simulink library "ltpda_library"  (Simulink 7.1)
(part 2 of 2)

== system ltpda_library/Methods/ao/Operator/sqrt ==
  In1 : Inport  OutDataType=sfix(16)  OutScaling=2^0
  sqrt : M-S-Function  Tag=sqrt  FunctionName=ltpdasim
  Out1 : Outport  OutDataType=sfix(16)  OutScaling=2^0
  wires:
  In1/1 -> sqrt/1
  sqrt/1 -> Out1/1

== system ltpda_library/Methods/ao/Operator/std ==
  In1 : Inport  OutDataType=sfix(16)  OutScaling=2^0
  std : M-S-Function  Tag=std  FunctionName=ltpdasim
  Out1 : Outport  OutDataType=sfix(16)  OutScaling=2^0
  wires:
  In1/1 -> std/1
  std/1 -> Out1/1

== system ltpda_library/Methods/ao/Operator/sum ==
  In1 : Inport  OutDataType=sfix(16)  OutScaling=2^0
  sum : M-S-Function  Tag=sum  FunctionName=ltpdasim
  Out1 : Outport  OutDataType=sfix(16)  OutScaling=2^0
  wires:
  In1/1 -> sum/1
  sum/1 -> Out1/1

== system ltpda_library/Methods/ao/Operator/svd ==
  In1 : Inport  OutDataType=sfix(16)  OutScaling=2^0
  svd : M-S-Function  Tag=svd  FunctionName=ltpdasim
  Out1 : Outport  OutDataType=sfix(16)  OutScaling=2^0
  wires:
  In1/1 -> svd/1
  svd/1 -> Out1/1

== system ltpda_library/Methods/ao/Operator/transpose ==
  In1 : Inport  OutDataType=sfix(16)  OutScaling=2^0
  transpose : M-S-Function  Tag=transpose  FunctionName=ltpdasim
  Out1 : Outport  OutDataType=sfix(16)  OutScaling=2^0
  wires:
  In1/1 -> transpose/1
  transpose/1 -> Out1/1

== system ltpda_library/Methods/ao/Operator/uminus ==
  In1 : Inport  OutDataType=sfix(16)  OutScaling=2^0
  uminus : M-S-Function  Tag=uminus  FunctionName=ltpdasim
  Out1 : Outport  OutDataType=sfix(16)  OutScaling=2^0
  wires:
  In1/1 -> uminus/1
  uminus/1 -> Out1/1

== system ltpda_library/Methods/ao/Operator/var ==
  In1 : Inport  OutDataType=sfix(16)  OutScaling=2^0
  var : M-S-Function  Tag=var  FunctionName=ltpdasim
  Out1 : Outport  OutDataType=sfix(16)  OutScaling=2^0
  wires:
  In1/1 -> var/1
  var/1 -> Out1/1

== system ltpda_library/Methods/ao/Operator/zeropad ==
  In1 : Inport  OutDataType=sfix(16)  OutScaling=2^0
  zeropad : M-S-Function  Tag=zeropad  FunctionName=ltpdasim
  Out1 : Outport  OutDataType=sfix(16)  OutScaling=2^0
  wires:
  In1/1 -> zeropad/1
  zeropad/1 -> Out1/1

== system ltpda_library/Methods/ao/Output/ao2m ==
  In1 : Inport  OutDataType=sfix(16)  OutScaling=2^0
  Terminator : Terminator
  ao2m : M-S-Function  Tag=ao2m  FunctionName=ltpdasim
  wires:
  ao2m/1 -> Terminator/1
  In1/1 -> ao2m/1

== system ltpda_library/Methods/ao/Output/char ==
  In1 : Inport  OutDataType=sfix(16)  OutScaling=2^0
  Terminator : Terminator
  char : M-S-Function  Tag=char  FunctionName=ltpdasim
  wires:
  char/1 -> Terminator/1
  In1/1 -> char/1

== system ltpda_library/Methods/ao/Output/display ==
  In1 : Inport  OutDataType=sfix(16)  OutScaling=2^0
  Terminator : Terminator
  display : M-S-Function  Tag=display  FunctionName=ltpdasim
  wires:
  display/1 -> Terminator/1
  In1/1 -> display/1

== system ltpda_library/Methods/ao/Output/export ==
  In1 : Inport  OutDataType=sfix(16)  OutScaling=2^0
  Terminator : Terminator
  export : M-S-Function  Tag=export  FunctionName=ltpdasim
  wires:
  export/1 -> Terminator/1
  In1/1 -> export/1

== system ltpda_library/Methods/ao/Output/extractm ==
  In1 : Inport  OutDataType=sfix(16)  OutScaling=2^0
  Terminator : Terminator
  extractm : M-S-Function  Tag=extractm  FunctionName=ltpdasim
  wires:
  extractm/1 -> Terminator/1
  In1/1 -> extractm/1

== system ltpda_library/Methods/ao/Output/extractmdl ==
  In1 : Inport  OutDataType=sfix(16)  OutScaling=2^0
  Terminator : Terminator
  extractmdl : M-S-Function  Tag=extractmdl  FunctionName=ltpdasim
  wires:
  extractmdl/1 -> Terminator/1
  In1/1 -> extractmdl/1

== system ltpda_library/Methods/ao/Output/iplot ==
  In1 : Inport  OutDataType=sfix(16)  OutScaling=2^0
  Terminator : Terminator
  iplot : M-S-Function  Tag=iplot  FunctionName=ltpdasim
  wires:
  iplot/1 -> Terminator/1
  In1/1 -> iplot/1

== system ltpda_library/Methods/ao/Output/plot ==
  In1 : Inport  OutDataType=sfix(16)  OutScaling=2^0
  Terminator : Terminator
  plot : M-S-Function  Tag=plot  FunctionName=ltpdasim
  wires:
  plot/1 -> Terminator/1
  In1/1 -> plot/1

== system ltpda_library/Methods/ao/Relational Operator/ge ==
  In1 : Inport  OutDataType=sfix(16)  OutScaling=2^0
  ge : M-S-Function  Tag=ge  FunctionName=ltpdasim
  Out1 : Outport  OutDataType=sfix(16)  OutScaling=2^0
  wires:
  In1/1 -> ge/1
  ge/1 -> Out1/1

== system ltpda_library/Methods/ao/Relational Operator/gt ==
  In1 : Inport  OutDataType=sfix(16)  OutScaling=2^0
  gt : M-S-Function  Tag=gt  FunctionName=ltpdasim
  Out1 : Outport  OutDataType=sfix(16)  OutScaling=2^0
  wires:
  In1/1 -> gt/1
  gt/1 -> Out1/1

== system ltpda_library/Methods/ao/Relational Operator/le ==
  In1 : Inport  OutDataType=sfix(16)  OutScaling=2^0
  le : M-S-Function  Tag=le  FunctionName=ltpdasim
  Out1 : Outport  OutDataType=sfix(16)  OutScaling=2^0
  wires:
  In1/1 -> le/1
  le/1 -> Out1/1

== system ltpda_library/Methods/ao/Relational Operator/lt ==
  In1 : Inport  OutDataType=sfix(16)  OutScaling=2^0
  lt : M-S-Function  Tag=lt  FunctionName=ltpdasim
  Out1 : Outport  OutDataType=sfix(16)  OutScaling=2^0
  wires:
  In1/1 -> lt/1
  lt/1 -> Out1/1

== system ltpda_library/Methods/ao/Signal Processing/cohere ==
  In1 : Inport  OutDataType=sfix(16)  OutScaling=2^0
  cohere : M-S-Function  Tag=cohere  FunctionName=ltpdasim
  Out1 : Outport  OutDataType=sfix(16)  OutScaling=2^0
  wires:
  In1/1 -> cohere/1
  cohere/1 -> Out1/1

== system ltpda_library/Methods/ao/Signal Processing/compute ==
  In1 : Inport  OutDataType=sfix(16)  OutScaling=2^0
  compute : M-S-Function  Tag=compute  FunctionName=ltpdasim
  Out1 : Outport  OutDataType=sfix(16)  OutScaling=2^0
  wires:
  In1/1 -> compute/1
  compute/1 -> Out1/1

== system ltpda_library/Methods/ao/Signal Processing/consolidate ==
  In1 : Inport  OutDataType=sfix(16)  OutScaling=2^0
  consolidate : M-S-Function  Tag=consolidate  FunctionName=ltpdasim
  Out1 : Outport  OutDataType=sfix(16)  OutScaling=2^0
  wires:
  In1/1 -> consolidate/1
  consolidate/1 -> Out1/1

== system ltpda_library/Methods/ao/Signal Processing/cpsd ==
  In1 : Inport  OutDataType=sfix(16)  OutScaling=2^0
  cpsd : M-S-Function  Tag=cpsd  FunctionName=ltpdasim
  Out1 : Outport  OutDataType=sfix(16)  OutScaling=2^0
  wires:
  In1/1 -> cpsd/1
  cpsd/1 -> Out1/1

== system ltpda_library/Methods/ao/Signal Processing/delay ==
  In1 : Inport  OutDataType=sfix(16)  OutScaling=2^0
  delay : M-S-Function  Tag=delay  FunctionName=ltpdasim
  Out1 : Outport  OutDataType=sfix(16)  OutScaling=2^0
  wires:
  In1/1 -> delay/1
  delay/1 -> Out1/1

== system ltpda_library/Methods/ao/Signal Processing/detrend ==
  In1 : Inport  OutDataType=sfix(16)  OutScaling=2^0
  detrend : M-S-Function  Tag=detrend  FunctionName=ltpdasim
  Out1 : Outport  OutDataType=sfix(16)  OutScaling=2^0
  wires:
  In1/1 -> detrend/1
  detrend/1 -> Out1/1

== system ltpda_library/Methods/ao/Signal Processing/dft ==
  In1 : Inport  OutDataType=sfix(16)  OutScaling=2^0
  dft : M-S-Function  Tag=dft  FunctionName=ltpdasim
  Out1 : Outport  OutDataType=sfix(16)  OutScaling=2^0
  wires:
  In1/1 -> dft/1
  dft/1 -> Out1/1

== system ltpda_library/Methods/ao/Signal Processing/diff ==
  In1 : Inport  OutDataType=sfix(16)  OutScaling=2^0
  diff : M-S-Function  Tag=diff  FunctionName=ltpdasim
  Out1 : Outport  OutDataType=sfix(16)  OutScaling=2^0
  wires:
  In1/1 -> diff/1
  diff/1 -> Out1/1

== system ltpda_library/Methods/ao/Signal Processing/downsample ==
  In1 : Inport  OutDataType=sfix(16)  OutScaling=2^0
  downsample : M-S-Function  Tag=downsample  FunctionName=ltpdasim
  Out1 : Outport  OutDataType=sfix(16)  OutScaling=2^0
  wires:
  In1/1 -> downsample/1
  downsample/1 -> Out1/1

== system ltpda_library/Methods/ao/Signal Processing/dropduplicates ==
  In1 : Inport  OutDataType=sfix(16)  OutScaling=2^0
  dropduplicates : M-S-Function  Tag=dropduplicates  FunctionName=ltpdasim
  Out1 : Outport  OutDataType=sfix(16)  OutScaling=2^0
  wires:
  In1/1 -> dropduplicates/1
  dropduplicates/1 -> Out1/1

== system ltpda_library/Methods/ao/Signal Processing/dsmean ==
  In1 : Inport  OutDataType=sfix(16)  OutScaling=2^0
  dsmean : M-S-Function  Tag=dsmean  FunctionName=ltpdasim
  Out1 : Outport  OutDataType=sfix(16)  OutScaling=2^0
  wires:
  In1/1 -> dsmean/1
  dsmean/1 -> Out1/1

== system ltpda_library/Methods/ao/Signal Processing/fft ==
  In1 : Inport  OutDataType=sfix(16)  OutScaling=2^0
  fft : M-S-Function  Tag=fft  FunctionName=ltpdasim
  Out1 : Outport  OutDataType=sfix(16)  OutScaling=2^0
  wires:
  In1/1 -> fft/1
  fft/1 -> Out1/1

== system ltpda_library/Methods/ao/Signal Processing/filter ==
  In1 : Inport  OutDataType=sfix(16)  OutScaling=2^0
  filter : M-S-Function  Tag=filter  FunctionName=ltpdasim
  Out1 : Outport  OutDataType=sfix(16)  OutScaling=2^0
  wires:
  In1/1 -> filter/1
  filter/1 -> Out1/1

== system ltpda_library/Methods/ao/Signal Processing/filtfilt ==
  In1 : Inport  OutDataType=sfix(16)  OutScaling=2^0
  filtfilt : M-S-Function  Tag=filtfilt  FunctionName=ltpdasim
  Out1 : Outport  OutDataType=sfix(16)  OutScaling=2^0
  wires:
  In1/1 -> filtfilt/1
  filtfilt/1 -> Out1/1

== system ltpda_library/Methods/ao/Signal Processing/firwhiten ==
  In1 : Inport  OutDataType=sfix(16)  OutScaling=2^0
  firwhiten : M-S-Function  Tag=firwhiten  FunctionName=ltpdasim
  Out1 : Outport  OutDataType=sfix(16)  OutScaling=2^0
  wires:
  In1/1 -> firwhiten/1
  firwhiten/1 -> Out1/1

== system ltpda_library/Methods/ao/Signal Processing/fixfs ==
  In1 : Inport  OutDataType=sfix(16)  OutScaling=2^0
  fixfs : M-S-Function  Tag=fixfs  FunctionName=ltpdasim
  Out1 : Outport  OutDataType=sfix(16)  OutScaling=2^0
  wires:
  In1/1 -> fixfs/1
  fixfs/1 -> Out1/1

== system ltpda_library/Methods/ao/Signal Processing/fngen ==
  In1 : Inport  OutDataType=sfix(16)  OutScaling=2^0
  fngen : M-S-Function  Tag=fngen  FunctionName=ltpdasim
  Out1 : Outport  OutDataType=sfix(16)  OutScaling=2^0
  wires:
  In1/1 -> fngen/1
  fngen/1 -> Out1/1

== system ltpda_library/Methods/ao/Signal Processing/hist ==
  In1 : Inport  OutDataType=sfix(16)  OutScaling=2^0
  hist : M-S-Function  Tag=hist  FunctionName=ltpdasim
  Out1 : Outport  OutDataType=sfix(16)  OutScaling=2^0
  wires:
  In1/1 -> hist/1
  hist/1 -> Out1/1

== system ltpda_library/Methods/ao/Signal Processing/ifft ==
  In1 : Inport  OutDataType=sfix(16)  OutScaling=2^0
  ifft : M-S-Function  Tag=ifft  FunctionName=ltpdasim
  Out1 : Outport  OutDataType=sfix(16)  OutScaling=2^0
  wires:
  In1/1 -> ifft/1
  ifft/1 -> Out1/1

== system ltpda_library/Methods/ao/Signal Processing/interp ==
  In1 : Inport  OutDataType=sfix(16)  OutScaling=2^0
  interp : M-S-Function  Tag=interp  FunctionName=ltpdasim
  Out1 : Outport  OutDataType=sfix(16)  OutScaling=2^0
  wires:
  In1/1 -> interp/1
  interp/1 -> Out1/1

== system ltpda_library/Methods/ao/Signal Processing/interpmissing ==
  In1 : Inport  OutDataType=sfix(16)  OutScaling=2^0
  interpmissing : M-S-Function  Tag=interpmissing  FunctionName=ltpdasim
  Out1 : Outport  OutDataType=sfix(16)  OutScaling=2^0
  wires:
  In1/1 -> interpmissing/1
  interpmissing/1 -> Out1/1

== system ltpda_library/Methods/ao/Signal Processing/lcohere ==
  In1 : Inport  OutDataType=sfix(16)  OutScaling=2^0
  lcohere : M-S-Function  Tag=lcohere  FunctionName=ltpdasim
  Out1 : Outport  OutDataType=sfix(16)  OutScaling=2^0
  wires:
  In1/1 -> lcohere/1
  lcohere/1 -> Out1/1

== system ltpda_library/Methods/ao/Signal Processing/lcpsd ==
  In1 : Inport  OutDataType=sfix(16)  OutScaling=2^0
  lcpsd : M-S-Function  Tag=lcpsd  FunctionName=ltpdasim
  Out1 : Outport  OutDataType=sfix(16)  OutScaling=2^0
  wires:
  In1/1 -> lcpsd/1
  lcpsd/1 -> Out1/1

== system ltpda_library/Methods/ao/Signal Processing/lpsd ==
  In1 : Inport  OutDataType=sfix(16)  OutScaling=2^0
  lpsd : M-S-Function  Tag=lpsd  FunctionName=ltpdasim
  Out1 : Outport  OutDataType=sfix(16)  OutScaling=2^0
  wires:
  In1/1 -> lpsd/1
  lpsd/1 -> Out1/1

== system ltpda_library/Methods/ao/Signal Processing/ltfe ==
  In1 : Inport  OutDataType=sfix(16)  OutScaling=2^0
  ltfe : M-S-Function  Tag=ltfe  FunctionName=ltpdasim
  Out1 : Outport  OutDataType=sfix(16)  OutScaling=2^0
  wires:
  In1/1 -> ltfe/1
  ltfe/1 -> Out1/1

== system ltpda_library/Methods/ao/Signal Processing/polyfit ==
  In1 : Inport  OutDataType=sfix(16)  OutScaling=2^0
  polyfit : M-S-Function  Tag=polyfit  FunctionName=ltpdasim
  Out1 : Outport  OutDataType=sfix(16)  OutScaling=2^0
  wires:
  In1/1 -> polyfit/1
  polyfit/1 -> Out1/1

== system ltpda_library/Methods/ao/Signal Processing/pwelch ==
  In1 : Inport  OutDataType=sfix(16)  OutScaling=2^0
  pwelch : M-S-Function  Tag=pwelch  FunctionName=ltpdasim
  Out1 : Outport  OutDataType=sfix(16)  OutScaling=2^0
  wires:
  In1/1 -> pwelch/1
  pwelch/1 -> Out1/1

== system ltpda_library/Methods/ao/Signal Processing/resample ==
  In1 : Inport  OutDataType=sfix(16)  OutScaling=2^0
  resample : M-S-Function  Tag=resample  FunctionName=ltpdasim
  Out1 : Outport  OutDataType=sfix(16)  OutScaling=2^0
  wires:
  In1/1 -> resample/1
  resample/1 -> Out1/1

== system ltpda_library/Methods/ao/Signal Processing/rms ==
  In1 : Inport  OutDataType=sfix(16)  OutScaling=2^0
  rms : M-S-Function  Tag=rms  FunctionName=ltpdasim
  Out1 : Outport  OutDataType=sfix(16)  OutScaling=2^0
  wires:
  In1/1 -> rms/1
  rms/1 -> Out1/1

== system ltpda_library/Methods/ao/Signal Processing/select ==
  In1 : Inport  OutDataType=sfix(16)  OutScaling=2^0
  select : M-S-Function  Tag=select  FunctionName=ltpdasim
  Out1 : Outport  OutDataType=sfix(16)  OutScaling=2^0
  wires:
  In1/1 -> select/1
  select/1 -> Out1/1

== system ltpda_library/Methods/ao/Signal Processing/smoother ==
  In1 : Inport  OutDataType=sfix(16)  OutScaling=2^0
  smoother : M-S-Function  Tag=smoother  FunctionName=ltpdasim
  Out1 : Outport  OutDataType=sfix(16)  OutScaling=2^0
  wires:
  In1/1 -> smoother/1
  smoother/1 -> Out1/1

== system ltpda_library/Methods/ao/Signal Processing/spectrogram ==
  In1 : Inport  OutDataType=sfix(16)  OutScaling=2^0
  spectrogram : M-S-Function  Tag=spectrogram  FunctionName=ltpdasim
  Out1 : Outport  OutDataType=sfix(16)  OutScaling=2^0
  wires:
  In1/1 -> spectrogram/1
  spectrogram/1 -> Out1/1

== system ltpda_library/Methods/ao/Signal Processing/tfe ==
  In1 : Inport  OutDataType=sfix(16)  OutScaling=2^0
  tfe : M-S-Function  Tag=tfe  FunctionName=ltpdasim
  Out1 : Outport  OutDataType=sfix(16)  OutScaling=2^0
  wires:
  In1/1 -> tfe/1
  tfe/1 -> Out1/1

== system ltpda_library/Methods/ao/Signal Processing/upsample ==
  In1 : Inport  OutDataType=sfix(16)  OutScaling=2^0
  upsample : M-S-Function  Tag=upsample  FunctionName=ltpdasim
  Out1 : Outport  OutDataType=sfix(16)  OutScaling=2^0
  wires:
  In1/1 -> upsample/1
  upsample/1 -> Out1/1

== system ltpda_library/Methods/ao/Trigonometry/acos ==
  In1 : Inport  OutDataType=sfix(16)  OutScaling=2^0
  acos : M-S-Function  Tag=acos  FunctionName=ltpdasim
  Out1 : Outport  OutDataType=sfix(16)  OutScaling=2^0
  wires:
  In1/1 -> acos/1
  acos/1 -> Out1/1

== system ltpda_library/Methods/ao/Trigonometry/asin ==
  In1 : Inport  OutDataType=sfix(16)  OutScaling=2^0
  asin : M-S-Function  Tag=asin  FunctionName=ltpdasim
  Out1 : Outport  OutDataType=sfix(16)  OutScaling=2^0
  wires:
  In1/1 -> asin/1
  asin/1 -> Out1/1

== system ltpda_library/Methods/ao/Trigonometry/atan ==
  In1 : Inport  OutDataType=sfix(16)  OutScaling=2^0
  atan : M-S-Function  Tag=atan  FunctionName=ltpdasim
  Out1 : Outport  OutDataType=sfix(16)  OutScaling=2^0
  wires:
  In1/1 -> atan/1
  atan/1 -> Out1/1

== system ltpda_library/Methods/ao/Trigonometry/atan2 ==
  In1 : Inport  OutDataType=sfix(16)  OutScaling=2^0
  atan2 : M-S-Function  Tag=atan2  FunctionName=ltpdasim
  Out1 : Outport  OutDataType=sfix(16)  OutScaling=2^0
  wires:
  In1/1 -> atan2/1
  atan2/1 -> Out1/1

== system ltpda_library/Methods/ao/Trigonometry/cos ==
  In1 : Inport  OutDataType=sfix(16)  OutScaling=2^0
  cos : M-S-Function  Tag=cos  FunctionName=ltpdasim
  Out1 : Outport  OutDataType=sfix(16)  OutScaling=2^0
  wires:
  In1/1 -> cos/1
  cos/1 -> Out1/1

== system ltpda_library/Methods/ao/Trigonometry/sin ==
  In1 : Inport  OutDataType=sfix(16)  OutScaling=2^0
  sin : M-S-Function  Tag=sin  FunctionName=ltpdasim
  Out1 : Outport  OutDataType=sfix(16)  OutScaling=2^0
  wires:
  In1/1 -> sin/1
  sin/1 -> Out1/1

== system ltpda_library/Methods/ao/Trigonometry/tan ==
  In1 : Inport  OutDataType=sfix(16)  OutScaling=2^0
  tan : M-S-Function  Tag=tan  FunctionName=ltpdasim
  Out1 : Outport  OutDataType=sfix(16)  OutScaling=2^0
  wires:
  In1/1 -> tan/1
  tan/1 -> Out1/1

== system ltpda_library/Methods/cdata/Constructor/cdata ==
  Ground : Ground
  cdata : M-S-Function  Tag=cdata  FunctionName=ltpdasim
  Out1 : Outport  OutDataType=sfix(16)  OutScaling=2^0
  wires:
  Ground/1 -> cdata/1
  cdata/1 -> Out1/1

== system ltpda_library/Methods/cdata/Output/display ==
  In1 : Inport  OutDataType=sfix(16)  OutScaling=2^0
  Terminator : Terminator
  display : M-S-Function  Tag=display  FunctionName=ltpdasim
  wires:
  display/1 -> Terminator/1
  In1/1 -> display/1

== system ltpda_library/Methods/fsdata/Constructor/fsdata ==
  Ground : Ground
  fsdata : M-S-Function  Tag=fsdata  FunctionName=ltpdasim
  Out1 : Outport  OutDataType=sfix(16)  OutScaling=2^0
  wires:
  Ground/1 -> fsdata/1
  fsdata/1 -> Out1/1

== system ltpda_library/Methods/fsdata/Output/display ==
  In1 : Inport  OutDataType=sfix(16)  OutScaling=2^0
  Terminator : Terminator
  display : M-S-Function  Tag=display  FunctionName=ltpdasim
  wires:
  display/1 -> Terminator/1
  In1/1 -> display/1

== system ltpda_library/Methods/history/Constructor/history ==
  Ground : Ground
  history : M-S-Function  Tag=history  FunctionName=ltpdasim
  Out1 : Outport  OutDataType=sfix(16)  OutScaling=2^0
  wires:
  Ground/1 -> history/1
  history/1 -> Out1/1

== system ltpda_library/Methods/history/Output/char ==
  In1 : Inport  OutDataType=sfix(16)  OutScaling=2^0
  Terminator : Terminator
  char : M-S-Function  Tag=char  FunctionName=ltpdasim
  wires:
  char/1 -> Terminator/1
  In1/1 -> char/1

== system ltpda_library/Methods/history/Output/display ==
  In1 : Inport  OutDataType=sfix(16)  OutScaling=2^0
  Terminator : Terminator
  display : M-S-Function  Tag=display  FunctionName=ltpdasim
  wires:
  display/1 -> Terminator/1
  In1/1 -> display/1

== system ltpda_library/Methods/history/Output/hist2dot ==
  In1 : Inport  OutDataType=sfix(16)  OutScaling=2^0
  Terminator : Terminator
  hist2dot : M-S-Function  Tag=hist2dot  FunctionName=ltpdasim
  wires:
  hist2dot/1 -> Terminator/1
  In1/1 -> hist2dot/1

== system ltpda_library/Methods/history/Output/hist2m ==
  In1 : Inport  OutDataType=sfix(16)  OutScaling=2^0
  Terminator : Terminator
  hist2m : M-S-Function  Tag=hist2m  FunctionName=ltpdasim
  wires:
  hist2m/1 -> Terminator/1
  In1/1 -> hist2m/1

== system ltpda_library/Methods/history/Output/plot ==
  In1 : Inport  OutDataType=sfix(16)  OutScaling=2^0
  Terminator : Terminator
  plot : M-S-Function  Tag=plot  FunctionName=ltpdasim
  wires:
  plot/1 -> Terminator/1
  In1/1 -> plot/1

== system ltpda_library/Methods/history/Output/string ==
  In1 : Inport  OutDataType=sfix(16)  OutScaling=2^0
  Terminator : Terminator
  string : M-S-Function  Tag=string  FunctionName=ltpdasim
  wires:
  string/1 -> Terminator/1
  In1/1 -> string/1

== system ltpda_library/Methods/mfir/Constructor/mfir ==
  Ground : Ground
  mfir : M-S-Function  Tag=mfir  FunctionName=ltpdasim
  Out1 : Outport  OutDataType=sfix(16)  OutScaling=2^0
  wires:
  Ground/1 -> mfir/1
  mfir/1 -> Out1/1

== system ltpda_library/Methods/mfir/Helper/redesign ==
  In1 : Inport  OutDataType=sfix(16)  OutScaling=2^0
  redesign : M-S-Function  Tag=redesign  FunctionName=ltpdasim
  Out1 : Outport  OutDataType=sfix(16)  OutScaling=2^0
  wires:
  In1/1 -> redesign/1
  redesign/1 -> Out1/1

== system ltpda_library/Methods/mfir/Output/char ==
  In1 : Inport  OutDataType=sfix(16)  OutScaling=2^0
  Terminator : Terminator
  char : M-S-Function  Tag=char  FunctionName=ltpdasim
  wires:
  char/1 -> Terminator/1
  In1/1 -> char/1

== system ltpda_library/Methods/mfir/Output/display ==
  In1 : Inport  OutDataType=sfix(16)  OutScaling=2^0
  Terminator : Terminator
  display : M-S-Function  Tag=display  FunctionName=ltpdasim
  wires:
  display/1 -> Terminator/1
  In1/1 -> display/1

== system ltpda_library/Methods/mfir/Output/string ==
  In1 : Inport  OutDataType=sfix(16)  OutScaling=2^0
  Terminator : Terminator
  string : M-S-Function  Tag=string  FunctionName=ltpdasim
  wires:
  string/1 -> Terminator/1
  In1/1 -> string/1

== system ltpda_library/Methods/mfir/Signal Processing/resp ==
  In1 : Inport  OutDataType=sfix(16)  OutScaling=2^0
  resp : M-S-Function  Tag=resp  FunctionName=ltpdasim
  Out1 : Outport  OutDataType=sfix(16)  OutScaling=2^0
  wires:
  In1/1 -> resp/1
  resp/1 -> Out1/1

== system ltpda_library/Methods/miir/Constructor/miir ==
  Ground : Ground
  miir : M-S-Function  Tag=miir  FunctionName=ltpdasim
  Out1 : Outport  OutDataType=sfix(16)  OutScaling=2^0
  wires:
  Ground/1 -> miir/1
  miir/1 -> Out1/1

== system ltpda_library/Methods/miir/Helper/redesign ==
  In1 : Inport  OutDataType=sfix(16)  OutScaling=2^0
  redesign : M-S-Function  Tag=redesign  FunctionName=ltpdasim
  Out1 : Outport  OutDataType=sfix(16)  OutScaling=2^0
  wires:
  In1/1 -> redesign/1
  redesign/1 -> Out1/1

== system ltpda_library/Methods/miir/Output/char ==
  In1 : Inport  OutDataType=sfix(16)  OutScaling=2^0
  Terminator : Terminator
  char : M-S-Function  Tag=char  FunctionName=ltpdasim
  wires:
  char/1 -> Terminator/1
  In1/1 -> char/1

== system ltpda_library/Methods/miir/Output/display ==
  In1 : Inport  OutDataType=sfix(16)  OutScaling=2^0
  Terminator : Terminator
  display : M-S-Function  Tag=display  FunctionName=ltpdasim
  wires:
  display/1 -> Terminator/1
  In1/1 -> display/1

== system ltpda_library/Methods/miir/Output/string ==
  In1 : Inport  OutDataType=sfix(16)  OutScaling=2^0
  Terminator : Terminator
  string : M-S-Function  Tag=string  FunctionName=ltpdasim
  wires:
  string/1 -> Terminator/1
  In1/1 -> string/1

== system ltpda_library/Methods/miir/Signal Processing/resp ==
  In1 : Inport  OutDataType=sfix(16)  OutScaling=2^0
  resp : M-S-Function  Tag=resp  FunctionName=ltpdasim
  Out1 : Outport  OutDataType=sfix(16)  OutScaling=2^0
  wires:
  In1/1 -> resp/1
  resp/1 -> Out1/1

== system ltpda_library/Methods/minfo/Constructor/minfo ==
  Ground : Ground
  minfo : M-S-Function  Tag=minfo  FunctionName=ltpdasim
  Out1 : Outport  OutDataType=sfix(16)  OutScaling=2^0
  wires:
  Ground/1 -> minfo/1
  minfo/1 -> Out1/1

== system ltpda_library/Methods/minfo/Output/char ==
  In1 : Inport  OutDataType=sfix(16)  OutScaling=2^0
  Terminator : Terminator
  char : M-S-Function  Tag=char  FunctionName=ltpdasim
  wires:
  char/1 -> Terminator/1
  In1/1 -> char/1

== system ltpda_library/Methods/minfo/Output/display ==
  In1 : Inport  OutDataType=sfix(16)  OutScaling=2^0
  Terminator : Terminator
  display : M-S-Function  Tag=display  FunctionName=ltpdasim
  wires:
  display/1 -> Terminator/1
  In1/1 -> display/1

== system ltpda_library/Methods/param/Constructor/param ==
  Ground : Ground
  param : M-S-Function  Tag=param  FunctionName=ltpdasim
  Out1 : Outport  OutDataType=sfix(16)  OutScaling=2^0
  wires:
  Ground/1 -> param/1
  param/1 -> Out1/1

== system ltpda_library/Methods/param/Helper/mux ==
  In1 : Inport  OutDataType=sfix(16)  OutScaling=2^0
  mux : M-S-Function  Tag=mux  FunctionName=ltpdasim
  Out1 : Outport  OutDataType=sfix(16)  OutScaling=2^0
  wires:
  In1/1 -> mux/1
  mux/1 -> Out1/1

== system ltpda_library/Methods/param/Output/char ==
  In1 : Inport  OutDataType=sfix(16)  OutScaling=2^0
  Terminator : Terminator
  char : M-S-Function  Tag=char  FunctionName=ltpdasim
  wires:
  char/1 -> Terminator/1
  In1/1 -> char/1

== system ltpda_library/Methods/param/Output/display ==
  In1 : Inport  OutDataType=sfix(16)  OutScaling=2^0
  Terminator : Terminator
  display : M-S-Function  Tag=display  FunctionName=ltpdasim
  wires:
  display/1 -> Terminator/1
  In1/1 -> display/1

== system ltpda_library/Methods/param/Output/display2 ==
  In1 : Inport  OutDataType=sfix(16)  OutScaling=2^0
  Terminator : Terminator
  display2 : M-S-Function  Tag=display2  FunctionName=ltpdasim
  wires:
  display2/1 -> Terminator/1
  In1/1 -> display2/1

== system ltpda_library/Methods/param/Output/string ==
  In1 : Inport  OutDataType=sfix(16)  OutScaling=2^0
  Terminator : Terminator
  string : M-S-Function  Tag=string  FunctionName=ltpdasim
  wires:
  string/1 -> Terminator/1
  In1/1 -> string/1

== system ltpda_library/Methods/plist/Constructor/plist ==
  Ground : Ground
  plist : M-S-Function  Tag=plist  FunctionName=ltpdasim
  Out1 : Outport  OutDataType=sfix(16)  OutScaling=2^0
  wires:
  Ground/1 -> plist/1
  plist/1 -> Out1/1

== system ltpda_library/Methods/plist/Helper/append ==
  In1 : Inport  OutDataType=sfix(16)  OutScaling=2^0
  append : M-S-Function  Tag=append  FunctionName=ltpdasim
  Out1 : Outport  OutDataType=sfix(16)  OutScaling=2^0
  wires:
  In1/1 -> append/1
  append/1 -> Out1/1

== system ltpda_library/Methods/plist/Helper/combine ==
  In1 : Inport  OutDataType=sfix(16)  OutScaling=2^0
  combine : M-S-Function  Tag=combine  FunctionName=ltpdasim
  Out1 : Outport  OutDataType=sfix(16)  OutScaling=2^0
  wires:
  In1/1 -> combine/1
  combine/1 -> Out1/1

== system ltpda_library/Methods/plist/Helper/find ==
  In1 : Inport  OutDataType=sfix(16)  OutScaling=2^0
  find : M-S-Function  Tag=find  FunctionName=ltpdasim
  Out1 : Outport  OutDataType=sfix(16)  OutScaling=2^0
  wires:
  In1/1 -> find/1
  find/1 -> Out1/1

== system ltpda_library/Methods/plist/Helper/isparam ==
  In1 : Inport  OutDataType=sfix(16)  OutScaling=2^0
  isparam : M-S-Function  Tag=isparam  FunctionName=ltpdasim
  Out1 : Outport  OutDataType=sfix(16)  OutScaling=2^0
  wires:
  In1/1 -> isparam/1
  isparam/1 -> Out1/1

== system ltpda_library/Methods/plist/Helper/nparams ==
  In1 : Inport  OutDataType=sfix(16)  OutScaling=2^0
  nparams : M-S-Function  Tag=nparams  FunctionName=ltpdasim
  Out1 : Outport  OutDataType=sfix(16)  OutScaling=2^0
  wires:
  In1/1 -> nparams/1
  nparams/1 -> Out1/1

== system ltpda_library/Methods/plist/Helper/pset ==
  In1 : Inport  OutDataType=sfix(16)  OutScaling=2^0
  pset : M-S-Function  Tag=pset  FunctionName=ltpdasim
  Out1 : Outport  OutDataType=sfix(16)  OutScaling=2^0
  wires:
  In1/1 -> pset/1
  pset/1 -> Out1/1

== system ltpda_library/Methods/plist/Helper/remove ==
  In1 : Inport  OutDataType=sfix(16)  OutScaling=2^0
  remove : M-S-Function  Tag=remove  FunctionName=ltpdasim
  Out1 : Outport  OutDataType=sfix(16)  OutScaling=2^0
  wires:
  In1/1 -> remove/1
  remove/1 -> Out1/1

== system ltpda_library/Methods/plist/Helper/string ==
  In1 : Inport  OutDataType=sfix(16)  OutScaling=2^0
  string : M-S-Function  Tag=string  FunctionName=ltpdasim
  Out1 : Outport  OutDataType=sfix(16)  OutScaling=2^0
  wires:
  In1/1 -> string/1
  string/1 -> Out1/1

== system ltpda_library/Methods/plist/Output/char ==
  In1 : Inport  OutDataType=sfix(16)  OutScaling=2^0
  Terminator : Terminator
  char : M-S-Function  Tag=char  FunctionName=ltpdasim
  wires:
  char/1 -> Terminator/1
  In1/1 -> char/1

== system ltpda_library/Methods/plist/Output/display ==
  In1 : Inport  OutDataType=sfix(16)  OutScaling=2^0
  Terminator : Terminator
  display : M-S-Function  Tag=display  FunctionName=ltpdasim
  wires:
  display/1 -> Terminator/1
  In1/1 -> display/1

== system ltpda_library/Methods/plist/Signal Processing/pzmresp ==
  In1 : Inport  OutDataType=sfix(16)  OutScaling=2^0
  pzmresp : M-S-Function  Tag=pzmresp  FunctionName=ltpdasim
  Out1 : Outport  OutDataType=sfix(16)  OutScaling=2^0
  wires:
  In1/1 -> pzmresp/1
  pzmresp/1 -> Out1/1

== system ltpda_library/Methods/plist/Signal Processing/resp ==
  In1 : Inport  OutDataType=sfix(16)  OutScaling=2^0
  resp : M-S-Function  Tag=resp  FunctionName=ltpdasim
  Out1 : Outport  OutDataType=sfix(16)  OutScaling=2^0
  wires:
  In1/1 -> resp/1
  resp/1 -> Out1/1

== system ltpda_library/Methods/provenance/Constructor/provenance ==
  Ground : Ground
  provenance : M-S-Function  Tag=provenance  FunctionName=ltpdasim
  Out1 : Outport  OutDataType=sfix(16)  OutScaling=2^0
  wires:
  Ground/1 -> provenance/1
  provenance/1 -> Out1/1

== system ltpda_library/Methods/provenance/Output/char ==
  In1 : Inport  OutDataType=sfix(16)  OutScaling=2^0
  Terminator : Terminator
  char : M-S-Function  Tag=char  FunctionName=ltpdasim
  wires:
  char/1 -> Terminator/1
  In1/1 -> char/1

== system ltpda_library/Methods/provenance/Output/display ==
  In1 : Inport  OutDataType=sfix(16)  OutScaling=2^0
  Terminator : Terminator
  display : M-S-Function  Tag=display  FunctionName=ltpdasim
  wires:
  display/1 -> Terminator/1
  In1/1 -> display/1

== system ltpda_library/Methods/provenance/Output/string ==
  In1 : Inport  OutDataType=sfix(16)  OutScaling=2^0
  Terminator : Terminator
  string : M-S-Function  Tag=string  FunctionName=ltpdasim
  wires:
  string/1 -> Terminator/1
  In1/1 -> string/1

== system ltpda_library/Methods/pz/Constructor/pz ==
  Ground : Ground
  pz : M-S-Function  Tag=pz  FunctionName=ltpdasim
  Out1 : Outport  OutDataType=sfix(16)  OutScaling=2^0
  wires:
  Ground/1 -> pz/1
  pz/1 -> Out1/1

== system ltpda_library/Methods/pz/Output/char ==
  In1 : Inport  OutDataType=sfix(16)  OutScaling=2^0
  Terminator : Terminator
  char : M-S-Function  Tag=char  FunctionName=ltpdasim
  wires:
  char/1 -> Terminator/1
  In1/1 -> char/1

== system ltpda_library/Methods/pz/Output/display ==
  In1 : Inport  OutDataType=sfix(16)  OutScaling=2^0
  Terminator : Terminator
  display : M-S-Function  Tag=display  FunctionName=ltpdasim
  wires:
  display/1 -> Terminator/1
  In1/1 -> display/1

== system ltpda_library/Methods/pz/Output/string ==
  In1 : Inport  OutDataType=sfix(16)  OutScaling=2^0
  Terminator : Terminator
  string : M-S-Function  Tag=string  FunctionName=ltpdasim
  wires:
  string/1 -> Terminator/1
  In1/1 -> string/1

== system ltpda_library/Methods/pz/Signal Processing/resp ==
  In1 : Inport  OutDataType=sfix(16)  OutScaling=2^0
  resp : M-S-Function  Tag=resp  FunctionName=ltpdasim
  Out1 : Outport  OutDataType=sfix(16)  OutScaling=2^0
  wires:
  In1/1 -> resp/1
  resp/1 -> Out1/1

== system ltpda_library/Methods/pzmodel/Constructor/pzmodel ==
  Ground : Ground
  pzmodel : M-S-Function  Tag=pzmodel  FunctionName=ltpdasim
  Out1 : Outport  OutDataType=sfix(16)  OutScaling=2^0
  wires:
  Ground/1 -> pzmodel/1
  pzmodel/1 -> Out1/1

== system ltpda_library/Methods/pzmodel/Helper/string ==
  In1 : Inport  OutDataType=sfix(16)  OutScaling=2^0
  string : M-S-Function  Tag=string  FunctionName=ltpdasim
  Out1 : Outport  OutDataType=sfix(16)  OutScaling=2^0
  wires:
  In1/1 -> string/1
  string/1 -> Out1/1

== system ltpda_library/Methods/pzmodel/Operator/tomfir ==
  In1 : Inport  OutDataType=sfix(16)  OutScaling=2^0
  tomfir : M-S-Function  Tag=tomfir  FunctionName=ltpdasim
  Out1 : Outport  OutDataType=sfix(16)  OutScaling=2^0
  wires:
  In1/1 -> tomfir/1
  tomfir/1 -> Out1/1

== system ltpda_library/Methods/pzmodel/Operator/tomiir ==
  In1 : Inport  OutDataType=sfix(16)  OutScaling=2^0
  tomiir : M-S-Function  Tag=tomiir  FunctionName=ltpdasim
  Out1 : Outport  OutDataType=sfix(16)  OutScaling=2^0
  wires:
  In1/1 -> tomiir/1
  tomiir/1 -> Out1/1

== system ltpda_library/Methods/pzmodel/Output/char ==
  In1 : Inport  OutDataType=sfix(16)  OutScaling=2^0
  Terminator : Terminator
  char : M-S-Function  Tag=char  FunctionName=ltpdasim
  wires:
  char/1 -> Terminator/1
  In1/1 -> char/1

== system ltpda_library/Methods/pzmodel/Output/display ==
  In1 : Inport  OutDataType=sfix(16)  OutScaling=2^0
  Terminator : Terminator
  display : M-S-Function  Tag=display  FunctionName=ltpdasim
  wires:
  display/1 -> Terminator/1
  In1/1 -> display/1

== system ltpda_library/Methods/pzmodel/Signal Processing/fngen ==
  In1 : Inport  OutDataType=sfix(16)  OutScaling=2^0
  fngen : M-S-Function  Tag=fngen  FunctionName=ltpdasim
  Out1 : Outport  OutDataType=sfix(16)  OutScaling=2^0
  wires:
  In1/1 -> fngen/1
  fngen/1 -> Out1/1

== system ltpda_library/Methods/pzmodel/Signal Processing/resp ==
  In1 : Inport  OutDataType=sfix(16)  OutScaling=2^0
  resp : M-S-Function  Tag=resp  FunctionName=ltpdasim
  Out1 : Outport  OutDataType=sfix(16)  OutScaling=2^0
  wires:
  In1/1 -> resp/1
  resp/1 -> Out1/1

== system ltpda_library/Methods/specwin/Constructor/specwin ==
  Ground : Ground
  specwin : M-S-Function  Tag=specwin  FunctionName=ltpdasim
  Out1 : Outport  OutDataType=sfix(16)  OutScaling=2^0
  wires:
  Ground/1 -> specwin/1
  specwin/1 -> Out1/1

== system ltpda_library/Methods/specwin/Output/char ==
  In1 : Inport  OutDataType=sfix(16)  OutScaling=2^0
  Terminator : Terminator
  char : M-S-Function  Tag=char  FunctionName=ltpdasim
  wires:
  char/1 -> Terminator/1
  In1/1 -> char/1

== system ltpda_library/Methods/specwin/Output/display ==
  In1 : Inport  OutDataType=sfix(16)  OutScaling=2^0
  Terminator : Terminator
  display : M-S-Function  Tag=display  FunctionName=ltpdasim
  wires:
  display/1 -> Terminator/1
  In1/1 -> display/1

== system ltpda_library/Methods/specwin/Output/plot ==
  In1 : Inport  OutDataType=sfix(16)  OutScaling=2^0
  Terminator : Terminator
  plot : M-S-Function  Tag=plot  FunctionName=ltpdasim
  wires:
  plot/1 -> Terminator/1
  In1/1 -> plot/1

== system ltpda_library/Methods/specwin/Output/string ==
  In1 : Inport  OutDataType=sfix(16)  OutScaling=2^0
  Terminator : Terminator
  string : M-S-Function  Tag=string  FunctionName=ltpdasim
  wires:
  string/1 -> Terminator/1
  In1/1 -> string/1

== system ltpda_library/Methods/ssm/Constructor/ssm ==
  Ground : Ground
  ssm : M-S-Function  Tag=ssm  FunctionName=ltpdasim
  Out1 : Outport  OutDataType=sfix(16)  OutScaling=2^0
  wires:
  Ground/1 -> ssm/1
  ssm/1 -> Out1/1

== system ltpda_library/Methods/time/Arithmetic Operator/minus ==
  In1 : Inport  OutDataType=sfix(16)  OutScaling=2^0
  minus : M-S-Function  Tag=minus  FunctionName=ltpdasim
  Out1 : Outport  OutDataType=sfix(16)  OutScaling=2^0
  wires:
  In1/1 -> minus/1
  minus/1 -> Out1/1

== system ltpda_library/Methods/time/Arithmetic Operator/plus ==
  In1 : Inport  OutDataType=sfix(16)  OutScaling=2^0
  plus : M-S-Function  Tag=plus  FunctionName=ltpdasim
  Out1 : Outport  OutDataType=sfix(16)  OutScaling=2^0
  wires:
  In1/1 -> plus/1
  plus/1 -> Out1/1

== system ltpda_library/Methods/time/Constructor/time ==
  Ground : Ground
  time : M-S-Function  Tag=time  FunctionName=ltpdasim
  Out1 : Outport  OutDataType=sfix(16)  OutScaling=2^0
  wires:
  Ground/1 -> time/1
  time/1 -> Out1/1

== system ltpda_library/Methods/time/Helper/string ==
  In1 : Inport  OutDataType=sfix(16)  OutScaling=2^0
  string : M-S-Function  Tag=string  FunctionName=ltpdasim
  Out1 : Outport  OutDataType=sfix(16)  OutScaling=2^0
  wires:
  In1/1 -> string/1
  string/1 -> Out1/1

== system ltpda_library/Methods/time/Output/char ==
  In1 : Inport  OutDataType=sfix(16)  OutScaling=2^0
  Terminator : Terminator
  char : M-S-Function  Tag=char  FunctionName=ltpdasim
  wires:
  char/1 -> Terminator/1
  In1/1 -> char/1

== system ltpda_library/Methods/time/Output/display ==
  In1 : Inport  OutDataType=sfix(16)  OutScaling=2^0
  Terminator : Terminator
  display : M-S-Function  Tag=display  FunctionName=ltpdasim
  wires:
  display/1 -> Terminator/1
  In1/1 -> display/1

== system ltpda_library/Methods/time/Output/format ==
  In1 : Inport  OutDataType=sfix(16)  OutScaling=2^0
  Terminator : Terminator
  format : M-S-Function  Tag=format  FunctionName=ltpdasim
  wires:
  format/1 -> Terminator/1
  In1/1 -> format/1

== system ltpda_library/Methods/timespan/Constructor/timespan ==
  Ground : Ground
  timespan : M-S-Function  Tag=timespan  FunctionName=ltpdasim
  Out1 : Outport  OutDataType=sfix(16)  OutScaling=2^0
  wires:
  Ground/1 -> timespan/1
  timespan/1 -> Out1/1

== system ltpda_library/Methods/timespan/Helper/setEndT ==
  In1 : Inport  OutDataType=sfix(16)  OutScaling=2^0
  setEndT : M-S-Function  Tag=setEndT  FunctionName=ltpdasim
  Out1 : Outport  OutDataType=sfix(16)  OutScaling=2^0
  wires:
  In1/1 -> setEndT/1
  setEndT/1 -> Out1/1

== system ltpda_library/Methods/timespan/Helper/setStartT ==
  In1 : Inport  OutDataType=sfix(16)  OutScaling=2^0
  setStartT : M-S-Function  Tag=setStartT  FunctionName=ltpdasim
  Out1 : Outport  OutDataType=sfix(16)  OutScaling=2^0
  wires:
  In1/1 -> setStartT/1
  setStartT/1 -> Out1/1

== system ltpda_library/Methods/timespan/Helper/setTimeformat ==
  In1 : Inport  OutDataType=sfix(16)  OutScaling=2^0
  setTimeformat : M-S-Function  Tag=setTimeformat  FunctionName=ltpdasim
  Out1 : Outport  OutDataType=sfix(16)  OutScaling=2^0
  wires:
  In1/1 -> setTimeformat/1
  setTimeformat/1 -> Out1/1

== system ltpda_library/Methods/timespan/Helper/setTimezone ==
  In1 : Inport  OutDataType=sfix(16)  OutScaling=2^0
  setTimezone : M-S-Function  Tag=setTimezone  FunctionName=ltpdasim
  Out1 : Outport  OutDataType=sfix(16)  OutScaling=2^0
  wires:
  In1/1 -> setTimezone/1
  setTimezone/1 -> Out1/1

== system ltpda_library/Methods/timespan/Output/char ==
  In1 : Inport  OutDataType=sfix(16)  OutScaling=2^0
  Terminator : Terminator
  char : M-S-Function  Tag=char  FunctionName=ltpdasim
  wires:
  char/1 -> Terminator/1
  In1/1 -> char/1

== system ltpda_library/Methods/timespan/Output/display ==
  In1 : Inport  OutDataType=sfix(16)  OutScaling=2^0
  Terminator : Terminator
  display : M-S-Function  Tag=display  FunctionName=ltpdasim
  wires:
  display/1 -> Terminator/1
  In1/1 -> display/1

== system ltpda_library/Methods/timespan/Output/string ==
  In1 : Inport  OutDataType=sfix(16)  OutScaling=2^0
  Terminator : Terminator
  string : M-S-Function  Tag=string  FunctionName=ltpdasim
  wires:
  string/1 -> Terminator/1
  In1/1 -> string/1

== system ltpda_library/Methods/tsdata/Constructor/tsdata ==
  Ground : Ground
  tsdata : M-S-Function  Tag=tsdata  FunctionName=ltpdasim
  Out1 : Outport  OutDataType=sfix(16)  OutScaling=2^0
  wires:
  Ground/1 -> tsdata/1
  tsdata/1 -> Out1/1

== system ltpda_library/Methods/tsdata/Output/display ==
  In1 : Inport  OutDataType=sfix(16)  OutScaling=2^0
  Terminator : Terminator
  display : M-S-Function  Tag=display  FunctionName=ltpdasim
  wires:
  display/1 -> Terminator/1
  In1/1 -> display/1

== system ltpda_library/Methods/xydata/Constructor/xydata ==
  Ground : Ground
  xydata : M-S-Function  Tag=xydata  FunctionName=ltpdasim
  Out1 : Outport  OutDataType=sfix(16)  OutScaling=2^0
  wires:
  Ground/1 -> xydata/1
  xydata/1 -> Out1/1

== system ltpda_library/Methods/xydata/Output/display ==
  In1 : Inport  OutDataType=sfix(16)  OutScaling=2^0
  Terminator : Terminator
  display : M-S-Function  Tag=display  FunctionName=ltpdasim
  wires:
  display/1 -> Terminator/1
  In1/1 -> display/1

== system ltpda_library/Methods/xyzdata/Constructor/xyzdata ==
  Ground : Ground
  xyzdata : M-S-Function  Tag=xyzdata  FunctionName=ltpdasim
  Out1 : Outport  OutDataType=sfix(16)  OutScaling=2^0
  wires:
  Ground/1 -> xyzdata/1
  xyzdata/1 -> Out1/1

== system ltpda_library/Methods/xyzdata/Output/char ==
  In1 : Inport  OutDataType=sfix(16)  OutScaling=2^0
  Terminator : Terminator
  char : M-S-Function  Tag=char  FunctionName=ltpdasim
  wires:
  char/1 -> Terminator/1
  In1/1 -> char/1

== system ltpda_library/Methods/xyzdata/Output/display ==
  In1 : Inport  OutDataType=sfix(16)  OutScaling=2^0
  Terminator : Terminator
  display : M-S-Function  Tag=display  FunctionName=ltpdasim
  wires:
  display/1 -> Terminator/1
  In1/1 -> display/1
